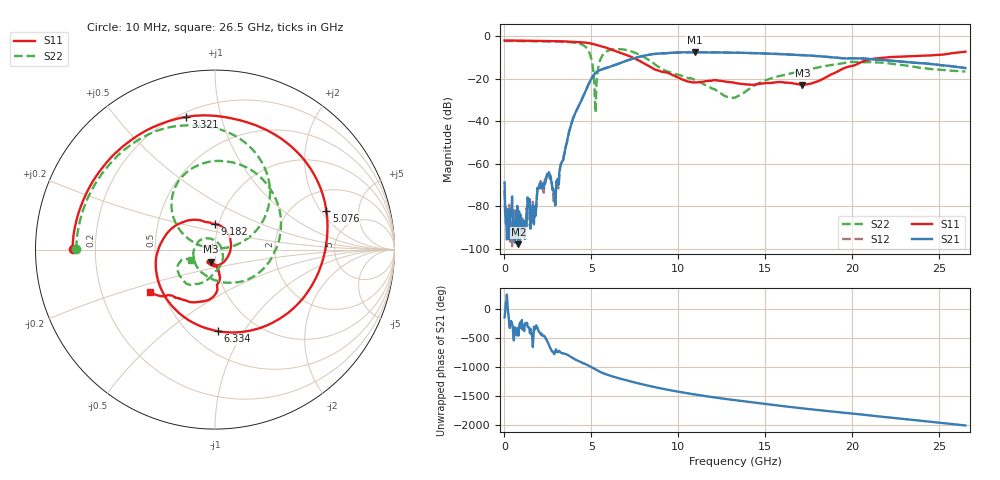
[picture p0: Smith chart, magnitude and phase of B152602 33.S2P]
!  2-Port S-parameters saved by WinCal
! VAR MeasName=S-Parameters (CALIBRATED_DATA) read from VNA (N5242A)
! VAR MeasDate=2016-1-5 16:31:00
! VAR NAME=B152602 33
! VAR FILENAME=B152602 33.S2P
! VAR DATE=2016-1-5 16:31:00
! VAR PHYS_PORTS=1,2
# Hz S DB R 50
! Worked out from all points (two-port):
!   801 points, 10 MHz to 26.5 GHz, reference 50 ohm
!   highest |S21| = -7.57 dB at 10.94 GHz (marker M1); lowest = -97.8 dB at 804.7 MHz (marker M2)
!   |S21| within 3 dB of the highest: 7.375 GHz to 20.73 GHz (13.36 GHz wide, 95 % of centre)
!   lowest |S11| = -22.9 dB at 17.13 GHz (marker M3), VSWR 1.15, Z = 47.3 - j6.44 ohm
!   |S11| at or under -10 dB: 7.353 GHz to 21.9 GHz (14.55 GHz wide, 99.5 % of centre)
!   |S22| runs from -36.0 to -2.2 dB; largest |S21 - S12| = 0.0028
!   S11 on the Smith chart (normalised r, x): 10 MHz: 0.12, +0.00; 3.321 GHz: 0.23, +0.78; 5.076 GHz: 2.98, +2.27; 6.334 GHz: 0.67, -0.77; 9.182 GHz: 0.96, +0.28; 26.5 GHz: 0.43, -0.25
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1e7  -2.02 179.8  -68.83 -140.2  -72.81 -110.9  -2.24 179.8
1.755625e8  -2.02 176.4  -90.95 85.3  -86.64 -100.5  -2.24 177.3
8.047e8  -2.09 163.5  -97.84 -94.0  -82.25 72.4  -2.28 167.6
1.698738e9  -2.20 144.7  -88.55 61.9  -79.98 46.6  -2.36 153.3
2.460325e9  -2.28 126.8  -64.67 170.4  -65.79 171.6  -2.44 139.9
2.890788e9  -2.34 115.3  -74.46 -18.5  -76.71 -26.1  -2.49 131.2
3.32125e9  -2.43 102.2  -58.88 -41.4  -58.60 -40.4  -2.59 121.1
4.447075e9  -2.88 57.4  -29.83 161.5  -29.82 161.6  -3.88 78.9
5.076212e9  -3.65 19.2  -18.94 68.8  -18.94 68.9  -14.18 19.0
5.274888e9  -4.07 5.4  -17.04 34.7  -17.03 34.9  -25.22 165.9
5.606012e9  -4.80 -20.4  -15.61 -13.9  -15.61 -13.6  -9.45 135.9
6.334488e9  -6.85 -88.2  -13.61 -89.5  -13.58 -89.4  -6.14 90.1
7.55965e9  -10.78 165.3  -10.13 172.1  -10.10 172.0  -7.97 22.9
8.851038e9  -16.18 102.8  -8.20 82.8  -8.21 82.7  -14.41 -74.2
9.182162e9  -16.95 89.5  -8.05 62.6  -8.06 62.7  -15.99 -102.2
1.093712e10  -21.79 -28.6  -7.57 -29.9  -7.58 -29.8  -20.54 143.0
1.3255e10  -21.97 -120.5  -7.76 -129.1  -7.75 -129.3  -28.89 8.0
1.491062e10  -22.17 -117.4  -8.15 168.1  -8.11 167.9  -21.15 -67.4
1.712916e10  -22.92 -108.6  -8.94 90.3  -8.92 90.5  -16.30 -98.2
1.769208e10  -22.10 -95.2  -9.20 71.3  -9.18 71.5  -15.29 -103.8
2.209604e10  -9.87 -114.2  -11.48 -67.0  -11.40 -67.2  -12.76 -155.1
2.65e10  -7.29 -146.6  -14.99 154.7  -14.98 154.3  -16.64 -156.2
